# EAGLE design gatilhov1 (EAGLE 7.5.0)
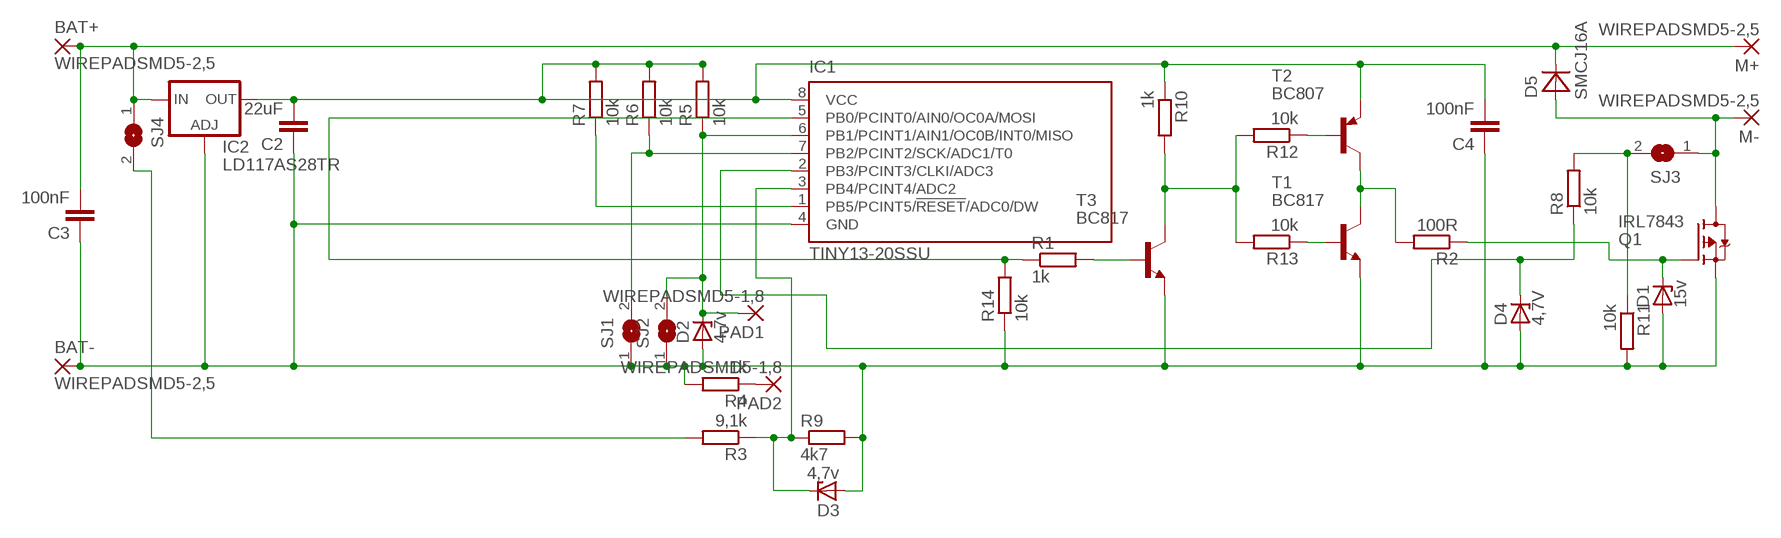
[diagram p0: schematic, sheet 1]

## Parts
BAT+  WIREPADSMD5-2,5  [5-2,5]
BAT-  WIREPADSMD5-2,5  [5-2,5]
C2  22uF  C-EUC1210K  [C1210K]
C3  100nF  C-EUC0805K  [C0805K]
C4  100nF  C-EUC1206K  [C1206K]
D1  15v  ZENER-DIODESOD80C  [SOD80C]
D2  4,7v  ZENER-DIODESOD80C  [SOD80C]
D3  4,7v  ZENER-DIODESOD80C  [SOD80C]
D4  4,7V  ZENER-DIODESOD80C  [SOD80C]
D5  SMCJ16A  MBRA340T3  [SMA]
IC1  TINY13-20SSU  [8S1]
IC2  LD117AS28TR  [SOT223]
M+  WIREPADSMD5-2,5  [5-2,5]
M-  WIREPADSMD5-2,5  [5-2,5]
PAD1  WIREPADSMD5-1,8  [5-1,8]
PAD2  WIREPADSMD5-1,8  [5-1,8]
Q1  IRL7843  FDD4141TO252  [TO252]
R1  1k  R-EU_R0805  [R0805]
R2  100R  R-EU_R0805  [R0805]
R3  9,1k  R-EU_R0805  [R0805]
R4  1k  R-EU_R0805  [R0805]
R5  10k  R-EU_R0805  [R0805]
R6  10k  R-EU_R0805  [R0805]
R7  10k  R-EU_R0805  [R0805]
R8  10k  R-EU_R0805  [R0805]
R9  4k7  R-EU_R0805  [R0805]
R10  1k  R-EU_R0805  [R0805]
R11  10k  R-EU_R0805  [R0805]
R12  10k  R-EU_R0805  [R0805]
R13  10k  R-EU_R0805  [R0805]
R14  10k  R-EU_R0805  [R0805]
SJ1  SJ  [SJ]
SJ2  SJ  [SJ]
SJ3  SJ  [SJ]
SJ4  SJ  [SJ]
T1  BC817  MMBT3904LT1-NPN-SOT23-BEC  [SOT23-BEC]
T2  BC807  MMBT3906LT1-PNP-SOT23-BEC  [SOT23-BEC]
T3  BC817  MMBT3904LT1-NPN-SOT23-BEC  [SOT23-BEC]

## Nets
N$1: BAT-.1(P) C2.1 C3.1 C4.1 D1.A D2.A D3.A D4.A IC1.4(GND) IC2.1(ADJ) Q1.2(S) R4.2 R9.2 R11.2 R14.1 SJ1.1 SJ2.1 T1.E T3.E
N$2: D5.A M-.1(P) Q1.3(D) SJ3.1
N$4: PAD2.1(P) R4.1
N$5: D4.C IC1.2(PB3/PCINT3/CLKI/ADC3) R8.1
N$6: IC1.5(PB0/PCINT0/AIN0/OC0A/MOSI) R1.1 R14.2
N$7: D2.C IC1.6(PB1/PCINT1/AIN1/OC0B/INT0/MISO) PAD1.1(P) R5.1 SJ2.2
N$8: D3.C IC1.3(PB4/PCINT4/ADC2) R3.1 R9.1
N$9: IC1.7(PB2/PCINT2/SCK/ADC1/T0) R6.1 SJ1.2
N$10: IC1.1(PB5/PCINT5/!RESET!/ADC0/DW) R7.1
N$11: R10.2 R12.2 R13.2 T3.C
N$12: R1.2 T3.B
N$13: R2.2 T1.C T2.C
N$14: BAT+.1(P) C3.2 D5.C IC2.3(IN) M+.1(P) SJ4.1
N$15: R12.1 T2.B
N$16: R13.1 T1.B
N$17: D1.C Q1.1(G) R2.1
N$18: R3.2 SJ4.2
N$19: R8.2 R11.1 SJ3.2
N$20: C2.2 C4.2 IC1.8(VCC) IC2.4(OUT) R5.2 R6.2 R7.2 R10.1 T2.E

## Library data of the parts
BAT+ BAT- M+ M- PAD1 PAD2 = wirepad:WIREPAD: Wire PAD connect wire on PCB
C2-C4 = rcl:C-EU: CAPACITOR, European symbol
D1-D4 = diode:ZENER-DIODE: Z-Diode
D5 = diode:MBRA340T3: Surface Mount Schottky Power Rectifier
IC1 = atmel:TINY13: 8-bit AVR Microcontroller with 1K Bytes In-System Programmable Flash Source: http://www.atmel.com/dyn/resources/prod_documents/2535S.pdf; MPN: ATTINY13-20SSU; OC_FARNELL: 1455133; OC_NEWARK: 58M3771
IC2 = v-reg:LD117A?*: Low drop fixed and adjustable positive voltage regulators 1 A Source: http://www.st.com/stonline/products/literature/ds/7194/ld1117axx.pdf
Q1 = transistor-fet:FDD4141: P-Channel PowerTrench® MOSFET Source: FDD4141.pdf
R1-R14 = resistor:R-EU_: RESISTOR, European symbol
SJ1-SJ4 = jumper:SJ: SMD solder JUMPER
T1 T3 = transistor-neu-to92:*-NPN-: NPN Transistror
T2 = transistor:*-PNP-: PNP Transistror

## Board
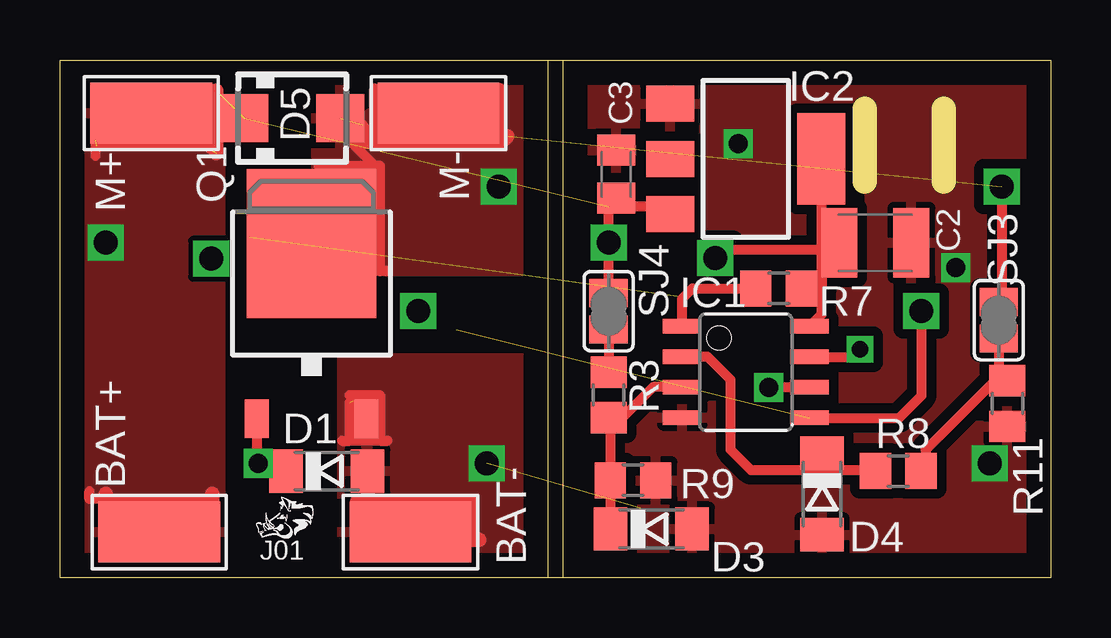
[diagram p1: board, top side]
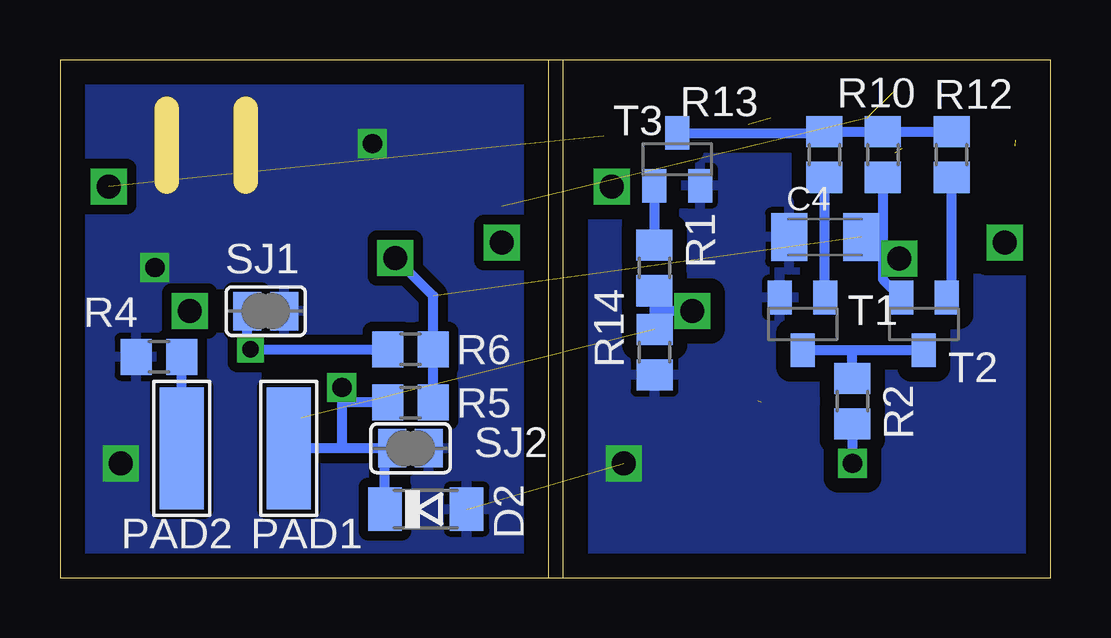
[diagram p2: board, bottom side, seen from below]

Size 41.27 x 21.59 mm. Coordinates in mm from the lower left corner, seen from the top.
Outline: 20.57,21.59 20.94,21.59 20.94,0
Outline: 20.33,21.59 20.33,0
Outline: 0,21.59 41.27,21.59 41.27,0 0,0 0,21.59
Copper layers (1*16): Top 0.035mm / dielectric 1.5mm / Bottom 0.035mm
Design rules "default": minimum track width 10mil, minimum drill 24mil, track to track 8mil, track to pad 8mil, pad to pad 8mil, via to via 8mil, smd to smd 8mil, copper to edge 40mil, drill to drill 8mil, minimum pad ring 10mil, minimum via ring 8mil, stop-mask expansion 4mil, vias tented up to drill 0mil, thermal gap 10mil
tRestrict: 2 lines
Milling: 2 lines

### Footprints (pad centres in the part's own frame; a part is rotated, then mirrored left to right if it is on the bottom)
5-2,5 = smd 2.54 x 5.08: 1 0,0
C1210K = smd 1.5 x 2.9: 1 -1.5,0; 2 1.5,0
C0805K = smd 1.3 x 1.6: 1 -1,0; 2 1,0
C1206K = smd 1.5 x 2: 1 -1.5,0; 2 1.5,0
SOD80C = smd 1.4 x 1.8: A 1.7,0; C -1.7,0
SMA = smd 2 x 2: A 2,0; C -2,0
8S1 = smd 0.6 x 1.6: 1 -1.905,-2.654; 2 -0.645,-2.654; 3 0.625,-2.654; 4 1.895,-2.654; 5 1.905,2.654; 6 0.635,2.654; 7 -0.635,2.654; 8 -1.905,2.654
SOT223 = smd 1.5 x 2: 1 -2.3,-3.15; 2 0,-3.15; 3 2.3,-3.15 | smd 3.8 x 2: 4 0,3.15
5-1,8 = smd 1.829 x 5.08: 1 0,0
TO252 = smd 1 x 1.6: 1 -2.28,-4.8; 2 2.28,-4.8 | smd 5.4 x 6.2: 3 0,2.5
R0805 = smd 1.3 x 1.5: 1 -0.95,0; 2 0.95,0
SJ = smd 1.168 x 1.6: 1 -0.762,0; 2 0.762,0
SOT23-BEC = smd 1 x 1.4: B -0.95,-1.1; C 0,1.1; E 0.95,-1.1

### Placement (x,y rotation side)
BAT+  4.13,1.91 90 top
BAT-  14.61,1.91 270 top
C2  33.97,13.97 180 top
C3  23.18,16.83 270 top
C4  9.4,14.2 0 bottom
D1  11.11,4.45 0 top
D2  26.04,2.86 0 bottom
D3  24.64,2.03 0 top
D4  31.75,3.49 270 top
D5  9.67,19.16 0 top
IC1  28.57,8.57 270 top
IC2  28.57,17.46 270 top
M+  3.81,19.37 90 top
M-  15.77,19.37 270 top
PAD1  31.75,5.4 0 bottom
PAD2  36.2,5.4 0 bottom
Q1  10.48,11.43 0 top
R1  16.51,12.92 90 bottom
R2  8.26,7.36 90 bottom
R3  22.86,7.62 90 top
R4  37.15,9.21 180 bottom
R5  26.67,7.3 0 bottom
R6  26.67,9.53 0 bottom
R7  29.95,12.07 0 top
R8  34.92,4.45 0 top
R9  23.88,4.06 0 top
R10  6.99,17.65 90 bottom
R11  39.47,7.26 270 top
R12  4.13,17.65 90 bottom
R13  9.43,17.65 90 bottom
R14  16.5,9.4 90 bottom
SJ1  32.7,11.11 180 bottom
SJ2  26.67,5.4 180 bottom
SJ3  39.12,10.74 270 top
SJ4  22.86,11.11 270 top
T1  10.33,10.58 180 bottom
T2  5.28,10.58 180 bottom
T3  15.56,17.45 0 bottom

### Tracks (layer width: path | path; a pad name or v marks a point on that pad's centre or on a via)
N$1  (via drill 0.8, 1)  (2 unrouted)
  Top 0.406: 13.34,5.71 13.65,5.71 | 12.06,7.62 13.34,7.62 13.34,5.71 | 13.34,5.71 12.06,5.71 | 12.06,5.71 12.06,7.3 | 11.75,5.71 12.06,5.71 | 12.19,7.37 12.19,7.11
  Top 0.61: 12.38,3.17 12.7,3.17 | 12.7,3.17 17.14,3.17 17.14,1.59 | D1.A 12.81,3.29 12.7,3.17 | 17.14,1.59 17.46,1.59 | 16.83,1.59 17.14,1.59
  other vias: 17.78,4.76 38.73,4.76 28.26,18.1 37.32,12.93
  pour Top: 11.75,0.32 19.37,0.32 19.37,9.14 11.75,9.14
  pour Top (isolate 0.406): 21.91,21.27 21.91,0.32 40.32,0.32 40.32,21.27
  pour Bottom (isolate 0.406): 40.32,21.27 40.32,0.32 21.91,0.32 21.91,21.27
  pour Bottom (isolate 0.61): 19.37,21.27 19.37,0.32 0.64,0.32 0.64,21.27
N$2  (via drill 1)  (2 unrouted)
  Top 0.406: 10.78,17.18 13.12,17.18 | 12.87,12.69 12.87,12.78 13.6,12.8 13.58,12.78 13.33,12.78 13.33,17.18 13.12,17.18 | 13.1,20.4 13.1,18.4 12.91,18.59 | v39.23,16.32 39.23,11.62 SJ3.1 | 13.12,17.18 12.2,18.1 13.3,18.1 | 12.91,18.41 12.91,18.59 | 12.91,18.59 12.6,18.9
  Top 0.61: 18.31,18.1 13.3,18.1 13.23,18.1 13.23,18.41 12.91,18.41 | 18.31,18.1 18.31,20.32 | 18.63,18.41 18.31,18.1
  other vias: 18.28,16.32
  pour Top: 10.66,21.27 10.64,12.78 19.37,12.78 19.37,21.27
N$4
  Bottom 0.406: PAD2.1 R4.1
N$5
  Top 0.406: IC1.2 26.98,9.22 27.94,8.26 27.94,5.33 28.78,4.49 31.7,4.49 | 31.7,4.49 33.93,4.49 R8.1 | D4.C 31.75,4.54 31.7,4.49
N$6  (via drill 1)  (1 unrouted)
  Top 0.406: IC1.5 34.97,6.67 35.9,7.6 35.9,11.09 v35.88,11.11
  Bottom 0.406: R1.1 16.51,11.1 | 16.51,11.1 R14.2 | v14.92,11.11 16.5,11.11 16.51,11.1
N$7  (via drill 0.8)
  Top 0.406: IC1.6 v29.53,7.94
  Bottom 0.406: v29.53,7.94 29.53,7.3 | 29.53,7.3 29.53,5.4 | R5.1 29.53,7.3 | 29.53,5.4 SJ2.2 27.73,5.09 D2.C | 29.53,5.4 PAD1.1
N$8
  Top 0.406: IC1.3 24.71,7.95 23.37,6.6 22.93,6.6 | 22.93,6.6 R3.1 | 22.93,6.6 R9.1 | R9.1 | D3.C R9.1
N$9  (via drill 0.7)
  Top 0.406: IC1.7 33.02,9.21 v33.34,9.53
  Bottom 0.406: R6.1 v33.34,9.53 33.47,9.53 SJ1.2
N$10
  Top 0.406: IC1.1 25.92,11.63 26.35,12.06 R7.1
N$11
  Bottom 0.406: 15.56,18.09 T3.C 9.38,18.55 R13.2 R10.2 R12.2
N$12
  Bottom 0.406: T3.B 16.51,13.97 R1.2
N$13
  Bottom 0.406: T2.C 8.3,9.48 | 8.3,9.48 T1.C | R2.2 8.26,9.44 8.3,9.48
N$14  (via drill 1)  (4 unrouted)
  Top 0.406: IC2.3 24.69,15.48 22.94,15.48 | 22.94,15.48 22.86,15.48 v22.86,13.97 SJ4.1 | 22.94,15.48 23.18,15.88 C3.2 | 1.77,18.25 1.47,18.25 1.47,17.59 | 2.23,3.29 1.22,3.29 1.22,3.61 | 1.5,18 6.2,18 6.2,17.9
  Top 0.61: 6.35,3.17 4.45,3.17 | 4.45,3.17 1.91,3.17 | BAT+.1 4.13,2.86 4.45,3.17 | 1.91,3.17 1.91,3.49 | 1.91,3.17 1.91,2.86 | 6.35,3.17 6.35,3.49 | 6.35,3.17 6.35,2.86 | 6.5,20.3 6.5,17.7
  other vias: 1.91,13.97
  pour Top: 0.64,0.32 0.64,21.27 6.67,21.27 6.67,0.32
N$15
  Bottom 0.406: R12.1 4.13,16.19 4.13,11.88 T2.B
N$16
  Bottom 0.406: R13.1 9.43,11.74 T1.B
N$17  (via drill 0.8)
  Top 0.406: Q1.1 8.2,4.82 v8.26,4.76 8.57,4.45 D1.C
  Bottom 0.406: R2.1 v8.26,4.76
N$18
  Top 0.406: SJ4.2 R3.2
N$19
  Top 0.406: 35.88,4.76 R8.2 36.07,4.64 36.07,5.33 38.95,8.21 R11.1 39.12,8.57 SJ3.2
N$20  (via drill 1)  (1 unrouted)
  Top 0.406: IC2.4 31.73,12.06 | 31.73,12.06 31.73,10.97 IC1.8 | 31.7,12.09 31.73,12.06 | R7.2 31.68,12.06 31.7,12.09 | 31.75,13.65 32.47,13.65 C2.2 | 31.75,13.65 27.62,13.65 v27.3,13.34 | 31.7,12.09 31.75,12.09 31.75,13.65
  Bottom 0.406: R5.2 R6.2 25.72,11.75 v27.3,13.34 | R10.1 6.99,14.2 | 6.99,14.2 6.99,13.3 | 6.99,13.3 6.99,12.44 T2.E | 6.99,13.3 v6.3,13.3 6.4,13.2 | C4.2 6.99,14.2

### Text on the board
tPlace: J01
